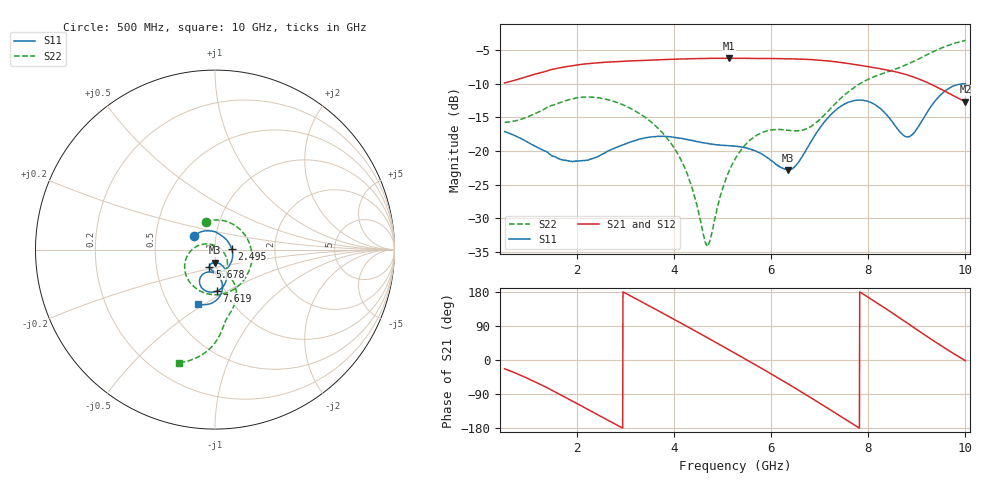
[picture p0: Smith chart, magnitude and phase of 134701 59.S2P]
!  2-Port S-parameters saved by WinCal
! VAR MeasName=S-Parameters (CALIBRATED_DATA) read from VNA (N5242A)
! VAR MeasDate=2013-7-3 16:40:58
! VAR NAME=134701 59
! VAR FILENAME=134701 59.S2P
! VAR DATE=2013-7-3 16:40:58
! VAR PHYS_PORTS=1,2
# Hz S MA R 50
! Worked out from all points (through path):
!   1601 points, 500 MHz to 10 GHz, reference 50 ohm
!   highest |S21| = -6.23 dB at 5.119 GHz (marker M1); lowest = -12.7 dB at 10 GHz (marker M2)
!   lowest |S11| = -22.8 dB at 6.343 GHz (marker M3), VSWR 1.16, Z = 49.6 - j7.2 ohm
!   |S11| at or under -10 dB: start of sweep to end of sweep
!   |S22| runs from -34.2 to -3.6 dB; largest |S21 - S12| = 0.0024
!   S11 on the Smith chart (normalised r, x): 500 MHz: 0.78, +0.12; 2.495 GHz: 1.21, +0.01; 5.678 GHz: 0.92, -0.18; 7.619 GHz: 0.91, -0.45; 10 GHz: 0.70, -0.47
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5e8  0.1393 147.0  0.3205 -23.1  0.3201 -23.1  0.1629 108.6
8.8e8  0.1214 122.1  0.3493 -43.1  0.3495 -43.0  0.1739 53.4
1.337188e9  0.0994 91.1  0.3893 -70.8  0.3896 -70.8  0.2062 -5.9
1.717188e9  0.08538 63.7  0.4192 -96.2  0.4196 -96.2  0.2334 -46.4
2.085312e9  0.08464 33.8  0.4395 -121.3  0.4396 -121.4  0.2506 -78.6
2.495e9  0.0939 1.4  0.4534 -149.6  0.4534 -149.7  0.2461 -108.5
3.082812e9  0.116 -40.9  0.4658 170.1  0.4659 170.1  0.2082 -142.8
3.670625e9  0.1284 -72.7  0.4759 129.7  0.4752 129.7  0.1465 -172.4
4.222812e9  0.1224 -92.5  0.4836 91.2  0.4833 91.2  0.07359 156.0
4.674062e9  0.1141 -100.1  0.4864 59.2  0.4869 59.3  0.01981 65.8
5.119375e9  0.1094 -103.6  0.4881 27.3  0.488 27.3  0.06959 -30.5
5.25e9  0.1084 -104.7  0.4876 17.8  0.488 17.8  0.08695 -39.6
5.6775e9  0.09981 -108.4  0.4863 -13.3  0.4873 -13.4  0.1293 -61.1
6.3425e9  0.07225 -89.0  0.484 -62.9  0.4845 -63.0  0.1422 -76.7
6.835312e9  0.1199 -62.9  0.4768 -101.4  0.4773 -101.3  0.1534 -66.5
7.256875e9  0.1907 -71.8  0.4618 -134.9  0.4626 -134.9  0.2132 -60.5
7.619062e9  0.2319 -87.6  0.444 -164.0  0.4451 -164.1  0.2807 -65.0
8.005e9  0.2322 -105.5  0.422 164.7  0.4226 164.6  0.342 -73.1
8.420625e9  0.1779 -117.8  0.397 130.2  0.3962 130.0  0.3893 -80.4
8.854062e9  0.1281 -95.1  0.3613 92.9  0.3617 92.7  0.4482 -85.0
9.418125e9  0.2449 -81.7  0.2972 44.5  0.2975 44.4  0.5634 -94.0
1e10  0.316 -107.1  0.2317 -1.9  0.2315 -2.1  0.6617 -107.8
